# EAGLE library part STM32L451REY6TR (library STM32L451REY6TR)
ARM Microcontrollers - MCU 16/32-BITS MICROS Source: Datasheet
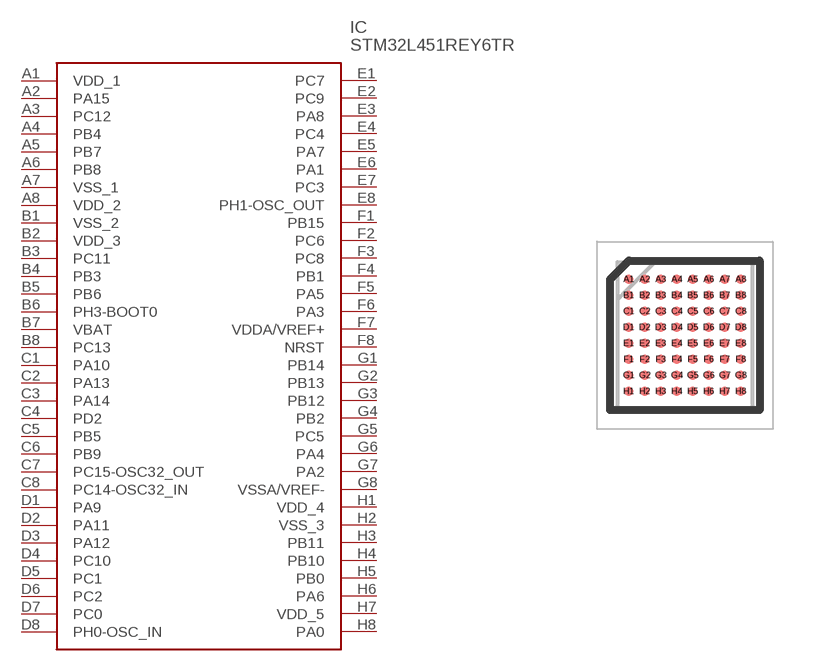
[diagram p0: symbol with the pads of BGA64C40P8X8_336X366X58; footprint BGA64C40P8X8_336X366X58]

Designator prefix IC

## STM32L451REY6TR (Arrow_Part_Number: STM32L451REY6TR; Arrow_Price-Stock: https://www.arrow.com/en/products/stm32l451rey6tr/stmicroelectronics?region=nac; Description: ARM Microcontrollers - MCU 16/32-BITS MICROS; Height: 0.585mm; Manufacturer_Name: STMicroelectronics; Manufacturer_Part_Number: STM32L451REY6TR; Mouser_Part_Number: 511-STM32L451REY6TR; Mouser_Price-Stock: https://www.mouser.co.uk/ProductDetail/STMicroelectronics/STM32L451REY6TR?qs=Mv7BduZupUg2YTQ5MbUYvA%3D%3D)  [BGA64C40P8X8_336X366X58]
A1  VDD_1
A2  PA15
A3  PC12
A4  PB4
A5  PB7
A6  PB8
A7  VSS_1
A8  VDD_2
B1  VSS_2
B2  VDD_3
B3  PC11
B4  PB3
B5  PB6
B6  PH3-BOOT0
B7  VBAT
B8  PC13
C1  PA10
C2  PA13
C3  PA14
C4  PD2
C5  PB5
C6  PB9
C7  PC15-OSC32_OUT
C8  PC14-OSC32_IN
D1  PA9
D2  PA11
D3  PA12
D4  PC10
D5  PC1
D6  PC2
D7  PC0
D8  PH0-OSC_IN
E1  PC7
E2  PC9
E3  PA8
E4  PC4
E5  PA7
E6  PA1
E7  PC3
E8  PH1-OSC_OUT
F1  PB15
F2  PC6
F3  PC8
F4  PB1
F5  PA5
F6  PA3
F7  VDDA/VREF+
F8  NRST
G1  PB14
G2  PB13
G3  PB12
G4  PB2
G5  PC5
G6  PA4
G7  PA2
G8  VSSA/VREF-
H1  VDD_4
H2  VSS_3
H3  PB11
H4  PB10
H5  PB0
H6  PA6
H7  VDD_5
H8  PA0

## Footprint BGA64C40P8X8_336X366X58 (pad centres in mm)
WLCSP - 64 balls, 3.357x3.657 mm 0.4 mm
smd 0.242 x 0.242: A1 -1.4,1.4; A2 -1,1.4; A3 -0.6,1.4; A4 -0.2,1.4; A5 0.2,1.4; A6 0.6,1.4; A7 1,1.4; A8 1.4,1.4; B1 -1.4,1; B2 -1,1; B3 -0.6,1; B4 -0.2,1; B5 0.2,1; B6 0.6,1; B7 1,1; B8 1.4,1; C1 -1.4,0.6; C2 -1,0.6; C3 -0.6,0.6; C4 -0.2,0.6; C5 0.2,0.6; C6 0.6,0.6; C7 1,0.6; C8 1.4,0.6; D1 -1.4,0.2; D2 -1,0.2; D3 -0.6,0.2; D4 -0.2,0.2; D5 0.2,0.2; D6 0.6,0.2; D7 1,0.2; D8 1.4,0.2; E1 -1.4,-0.2; E2 -1,-0.2; E3 -0.6,-0.2; E4 -0.2,-0.2; E5 0.2,-0.2; E6 0.6,-0.2; E7 1,-0.2; E8 1.4,-0.2; F1 -1.4,-0.6; F2 -1,-0.6; F3 -0.6,-0.6; F4 -0.2,-0.6; F5 0.2,-0.6; F6 0.6,-0.6; F7 1,-0.6; F8 1.4,-0.6; G1 -1.4,-1; G2 -1,-1; G3 -0.6,-1; G4 -0.2,-1; G5 0.2,-1; G6 0.6,-1; G7 1,-1; G8 1.4,-1; H1 -1.4,-1.4; H2 -1,-1.4; H3 -0.6,-1.4; H4 -0.2,-1.4; H5 0.2,-1.4; H6 0.6,-1.4; H7 1,-1.4; H8 1.4,-1.4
